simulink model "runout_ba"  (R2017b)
settings: Solver=VariableStepAuto  StartTime=0.0  StopTime=10.0  RelTol=1e-3

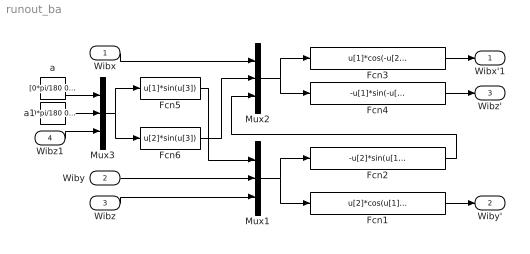
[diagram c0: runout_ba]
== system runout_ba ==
  Wibx : Inport
  Wiby : Inport  Port=2
  Wibz : Inport  Port=3
  Wibz1 : Inport  Port=4
  Fcn1 : Fcn  Expr=u[2]*cos(u[1])+u[3]*sin(u[1])
  Fcn2 : Fcn  Expr=-u[2]*sin(u[1])+u[3]*cos(u[1])
  Fcn3 : Fcn  Expr=u[1]*cos(-u[2])+u[3]*sin(-u[2])
  Fcn4 : Fcn  Expr=-u[1]*sin(-u[2])+u[3]*cos(-u[2])
  Fcn5 : Fcn  Expr=u[1]*sin(u[3])
  Fcn6 : Fcn  Expr=u[2]*sin(u[3])
  Mux1 : Mux  Inputs=3
  Mux2 : Mux  Inputs=3
  Mux3 : Mux  Inputs=3
  a : Constant  Value=[0*pi/180 0*pi/180 0*pi/180]'
  a1 : Constant  Value=[0*pi/180 0*pi/180 0*pi/180]'
  Wibx'1 : Outport
  Wiby' : Outport  Port=2
  Wibz' : Outport  Port=3
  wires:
  Mux2/1 -> Fcn3/1, Fcn4/1
  Fcn6/1 -> Mux2/2
  Fcn4/1 -> Wibz'/1
  Wibx/1 -> Mux2/1
  Wibz/1 -> Mux1/3
  Mux1/1 -> Fcn1/1, Fcn2/1
  Fcn3/1 -> Wibx'1/1
  Wiby/1 -> Mux1/2
  Fcn5/1 -> Mux1/1
  Fcn2/1 -> Mux2/3
  Fcn1/1 -> Wiby'/1
  a/1 -> Mux3/1
  a1/1 -> Mux3/2
  Wibz1/1 -> Mux3/3
  Mux3/1 -> Fcn6/1, Fcn5/1
